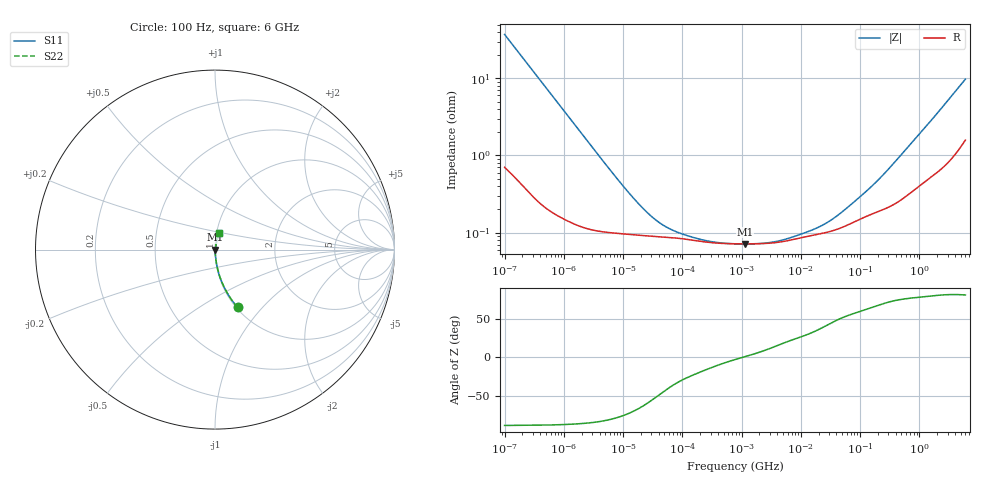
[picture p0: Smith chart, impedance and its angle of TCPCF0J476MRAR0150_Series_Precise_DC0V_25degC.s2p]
! TCPCF0J476MRAR0150 Polymer Tantalum Capacitor Sparameter Model
! Model Generated by Samsung Electro-Mechanics
! Samsung Sparameter Version 5.0
! Date : Oct-21-2025
! Products : Polymer Tantalum Capacitor
! Characteristics :
!  Nominal Capacitance = 47uF
!  Capacitance Tolerance = +/-20%
!  ESR = 150 mohm max at 100kHz
!  Rated Voltage = 6.3Vdc
!  Size = 0805(unit:inch), 2012(unit:mm)
!  Length = 2.00+/-0.20mm
!  Width = 1.25+/-0.20mm
!  Thickness = 0.90+/-0.10mm
!  Lineup = Conductive Polymer Type
!  Feature = PCF
!  Measurement Temperature : 25degC.
!  DC bias Value = 0V
!  Frequency : 100Hz ~ 6GHz
! External Node Assignments :
!  1  o---||---o  2
# MHz S RI R 50.0
! Freq.  Real(S11)  Im(S11)  Real(S12)  Im(S12)  Real(S21)  Im(S21)  Real(S22)  Im(S22)
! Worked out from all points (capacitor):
!   300 points, 100 Hz to 6 GHz, reference 50 ohm
!   read as one part in series: C = 42.7 uF near 106.2 Hz
!   lowest |Z| = 71.3 mohm at 1.143 MHz (marker M1)
!   series resonance near 1.088 MHz, so ESL is about 500 pH
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0.0001  0.1258 -0.3223  0.8742 0.3223  0.8742 0.3223  0.1258 -0.3223
0.0001714451  0.0494 -0.2062  0.9506 0.2062  0.9506 0.2062  0.0494 -0.2062
0.0003517965  0.0138 -0.1053  0.9862 0.1053  0.9862 0.1053  0.0138 -0.1053
0.0007664292  0.0041 -0.0492  0.9959 0.0492  0.9959 0.0492  0.0041 -0.0492
0.001998454  0.00155 -0.0191  0.9985 0.0191  0.9985 0.0191  0.00155 -0.0191
0.01358747  0.00095 -0.00289  0.9991 0.00289  0.9991 0.00289  0.00095 -0.00289
0.02473303  0.000909 -0.00162  0.9991 0.00162  0.9991 0.00162  0.000909 -0.00162
0.03993819  0.000885 -0.00104  0.9991 0.00104  0.9991 0.00104  0.000885 -0.00104
0.0726988  0.000854 -0.000614  0.9991 0.000614  0.9991 0.000614  0.000854 -0.000614
0.1583827  0.000791 -0.000332  0.9992 0.000332  0.9992 0.000332  0.000791 -0.000332
0.3450549  0.000735 -0.000161  0.9993 0.000161  0.9993 0.000161  0.000735 -0.000161
0.7981464  0.000714 -3.76e-05  0.9993 3.76e-05  0.9993 3.76e-05  0.000714 -3.76e-05
1.143315  0.000712 6.04e-06  0.9993 -6.04e-06  0.9993 -6.04e-06  0.000712 6.04e-06
2.346024  0.00072 0.000102  0.9993 -0.000102  0.9993 -0.000102  0.00072 0.000102
4.022142  0.000745 0.000199  0.9993 -0.000199  0.9993 -0.000199  0.000745 0.000199
15.95059  0.000921 0.00058  0.9991 -0.00058  0.9991 -0.00058  0.000921 0.00058
27.3465  0.00101 0.000878  0.999 -0.000878  0.999 -0.000878  0.00101 0.000878
49.77836  0.00117 0.00144  0.9988 -0.00144  0.9988 -0.00144  0.00117 0.00144
146.3155  0.0017 0.00337  0.9983 -0.00337  0.9983 -0.00337  0.0017 0.00337
318.7652  0.00222 0.00659  0.9978 -0.00659  0.9978 -0.00659  0.00222 0.00659
1922.593  0.00694 0.033  0.9931 -0.033  0.9931 -0.033  0.00694 0.033
6000  0.0244 0.0926  0.9756 -0.0926  0.9756 -0.0926  0.0244 0.0926
